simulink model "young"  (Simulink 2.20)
settings: Solver=ode45  StartTime=0.0  StopTime=10.0  RelTol=1e-3  AbsTol=1e-6
libraries: simulink x1

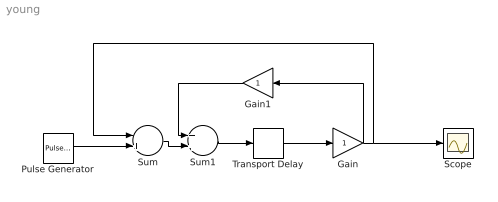
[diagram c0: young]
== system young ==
  Gain : Gain  Gain=1
  Gain1 : Gain  Orientation=left  Gain=1
  Pulse Generator : simulink/Sources/Pulse Generator  period=1000  duty=50  amplitude=20  start=2
  Scope : Scope
  Sum : Sum  Inputs=-+
  Sum1 : Sum  Inputs=++
  Transport Delay : TransportDelay  DelayTime=.07  InitialInput=0  BufferSize=1024
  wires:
  Pulse Generator/1 -> Sum/2
  Sum/1 -> Sum1/2
  Sum1/1 -> Transport Delay/1
  Transport Delay/1 -> Gain/1
  Gain/1 -> Scope/1, Sum/1, Gain1/1
  Gain1/1 -> Sum1/1
